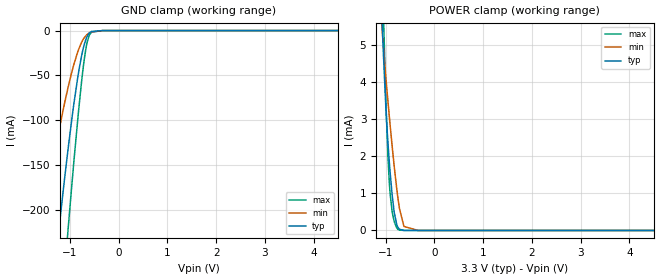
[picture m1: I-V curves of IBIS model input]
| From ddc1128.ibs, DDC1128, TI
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|   input Model
[Model]   input
Model_type   Input
Vinl = 0.66
Vinh = 2.64
|   typ   min   max
|   (nom PVT)   (fast PVT)   (slow PVT)
C_comp   7.024e-12   5.695e-12   8.472e-12
[Model spec]
|Subparameter
Vinl   0.66   0.54   0.72
Vinh   2.64   2.16   2.88
| Where nom  PVT is Nominal Process, 3.3V, 27C
|   Fast PVT is Strong Process,  3.6V, -40C
|   Slow PVT is Weak Process,   2.7V, 125C
[Voltage Range]   3.3   2.7   3.6
|Junction Temperature
[Temperature Range]   27   125   -40
[Power Clamp Reference]   3.3   2.7   3.6
[GND Clamp Reference]   0   0   0
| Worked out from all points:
|   GND clamp passes 1 mA (typ) near -0.56 V on its own axis
|   POWER clamp passes 1 mA (typ) near -0.87 V on its own axis
[GND Clamp]
|   Voltage   I(typ)   I(min)   I(max)
-3.3V     -1.457A    -942.6mA   -1.834A
-1.777V   -527.4mA   -294.2mA   -742mA
-1.482V   -358.6mA   -190.5mA   -530.1mA
-1.251V   -235mA     -119.2mA   -366.8mA
-1.165V   -192mA     -95.41mA   -307.5mA
-1.033V   -130mA     -62.28mA   -218.8mA
-930.6mV  -86.47mA   -40.09mA   -153.6mA
-837.6mV  -51.78mA   -23.49mA   -98.39mA
-732.6mV  -21.27mA   -10.34mA   -43.74mA
-643.2mV  -6.113mA   -4.238mA   -12.41mA
-556.8mV  -993.6uA   -1.536mA   -1.699mA
6.6V      0A         0A         0A
[POWER Clamp]
|   Voltage   I(typ)   I(min)   I(max)
-3.3V     121.5mA    94.93mA    149.3mA
-1.069V   5.467mA    5.301mA    6.937mA
-1.046V   4.694mA    4.901mA    5.765mA
-999.6mV  3.349mA    4.144mA    3.595mA
-956.4mV  2.381mA    3.493mA    2.023mA
-910.8mV  1.565mA    2.841mA    985uA
-826.8mV  488.3uA    1.729mA    239.8uA
-772.8mV  148.8uA    1.102mA    61.39uA
-719.4mV  32.85uA    595uA      10.31uA
-627mV    1.959uA    107.2uA    477.3nA
-330mV    0A         36.85nA    0A
6.6V      0A         0A         0A
